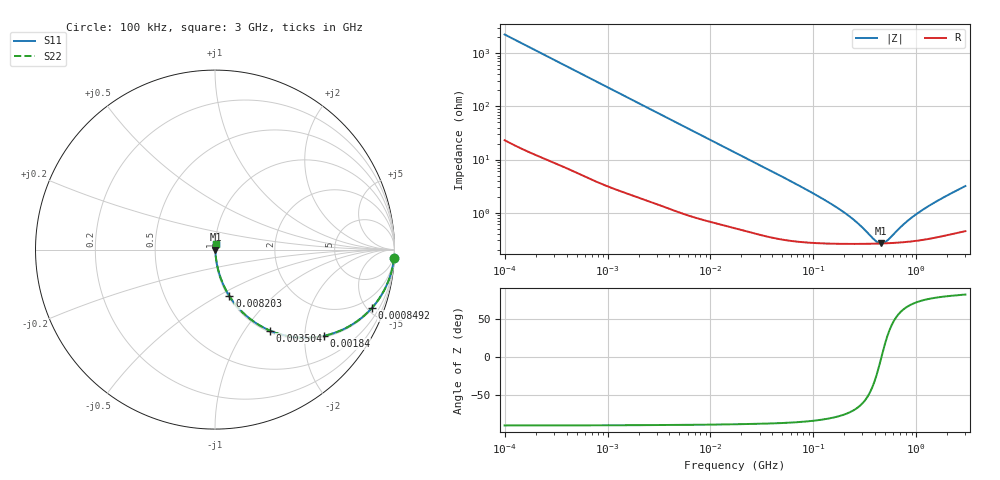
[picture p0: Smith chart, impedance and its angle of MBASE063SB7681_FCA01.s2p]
! MBASE063SB7681_FCA01  S-PARAMETER MODEL  ( Standard Model )
! Model Generated by TAIYO YUDEN Corporation (http://www.ty-top.com)
! Version 2.0
! TAIYO YUDEN Control No. 231201
! Copyright(c) 2022 TAIYO YUDEN CO.,LTD. All Rights Reserved.
! Product Description (link to TY-COMPAS)
! https://ds.yuden.co.jp/TYCOMPAS/or/detail?pn=MBASE063SB7681KFCA01&u=M
! Products Name : Multilayer Ceramic Capacitors
! Characteristics :
!  Capacitance : 680 [pF] , Rated Voltage : 16 [V] , TCC : X7R
!  Case Size : 0.6 x 0.3 / 0.024 x 0.012 [mm/inch] , Thickness : 0.3 / 0.012 [mm/inch]
!  (Conditions: Temperature = 25 [degC] , DC Bias Voltage = 0 [V])
! External Node Assignments :
!  1  o---| |---o  2
! GND o---------o GND
! Frequency Range : 100kHz  -  3GHz  [ 401 STEP ]
# MHZ S RI R 50
! Freq[MHz].  S11 Real  S11 Imag  S21 Real  S21 Imag  S12 Real  S12 Imag  S22 Real  S22 Imag
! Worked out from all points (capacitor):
!   401 points, 100 kHz to 3 GHz, reference 50 ohm
!   read as one part in series: C = 706 pF near 105.3 kHz
!   lowest |Z| = 263 mohm at 457.1 MHz (marker M1)
!   series resonance near 458.4 MHz, so ESL is about 170 pH
!   S11 on the Smith chart (normalised r, x): 100 kHz: 1, -45; 849.2 kHz: 1.07, -5.37; 1.84 MHz: 1.04, -2.50; 3.504 MHz: 1.03, -1.32; 8.203 MHz: 1.01, -0.57; 3 GHz: 1.01, +0.06
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0.1  0.9976 -0.0443  0.00242 0.0443  0.00242 0.0443  0.9976 -0.0443
0.259498  0.9858 -0.1129  0.0142 0.1129  0.0142 0.1129  0.9858 -0.1129
0.562235  0.9399 -0.2315  0.0601 0.2315  0.0601 0.2315  0.9399 -0.2315
0.849186  0.8751 -0.324  0.1249 0.324  0.1249 0.324  0.8751 -0.324
1.249956  0.767 -0.4156  0.233 0.4156  0.233 0.4156  0.767 -0.4156
1.839868  0.6072 -0.4803  0.3928 0.4803  0.3928 0.4803  0.6072 -0.4803
3.161081  0.3506 -0.4677  0.6494 0.4677  0.6494 0.4677  0.3506 -0.4677
3.504345  0.3067 -0.4514  0.6933 0.4514  0.6933 0.4514  0.3067 -0.4514
5.292876  0.1667 -0.3618  0.8333 0.3618  0.8333 0.3618  0.1667 -0.3618
8.202936  0.0805 -0.2593  0.9195 0.2593  0.9195 0.2593  0.0805 -0.2593
17.7727  0.022 -0.1288  0.978 0.1288  0.978 0.1288  0.022 -0.1288
37.52708  0.00738 -0.0624  0.9926 0.0624  0.9926 0.0624  0.00738 -0.0624
97.38194  0.00324 -0.0234  0.9968 0.0234  0.9968 0.0234  0.00324 -0.0234
210.9903  0.00266 -0.00891  0.9973 0.00891  0.9973 0.00891  0.00266 -0.00891
280.1453  0.00261 -0.00533  0.9974 0.00533  0.9974 0.00533  0.00261 -0.00533
401.8672  0.00261 -0.00137  0.9974 0.00137  0.9974 0.00137  0.00261 -0.00137
457.1373  0.00263 -2.92e-05  0.9974 2.92e-05  0.9974 2.92e-05  0.00263 -2.92e-05
547.5153  0.00267 0.00185  0.9973 -0.00185  0.9973 -0.00185  0.00267 0.00185
765.4251  0.00282 0.00553  0.9972 -0.00553  0.9972 -0.00553  0.00282 0.00553
1070.062  0.0031 0.00977  0.9969 -0.00977  0.9969 -0.00977  0.0031 0.00977
1701.687  0.00382 0.0173  0.9962 -0.0173  0.9962 -0.0173  0.00382 0.0173
3000  0.00545 0.0311  0.9946 -0.0311  0.9946 -0.0311  0.00545 0.0311
